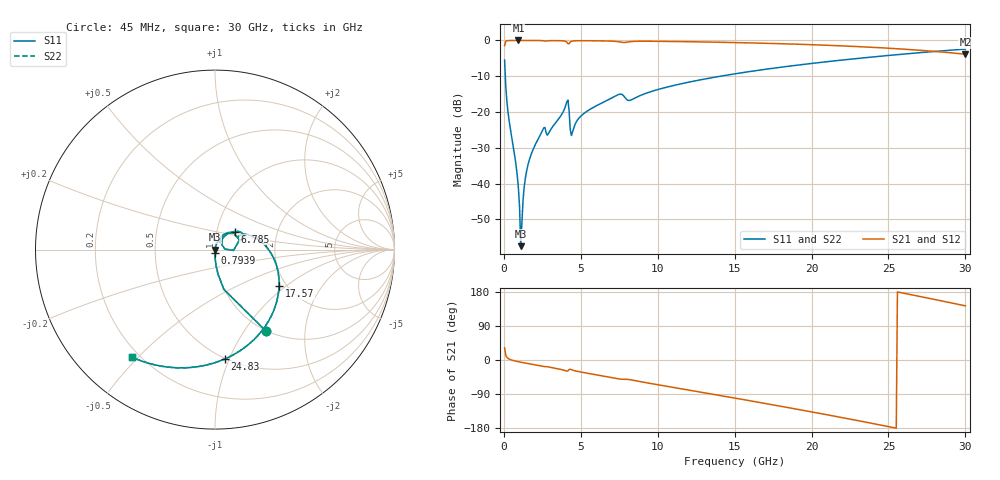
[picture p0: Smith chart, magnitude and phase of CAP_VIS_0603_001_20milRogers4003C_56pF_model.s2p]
! S-parameter model data by Modelithics Inc.  support@modelithics.com  813-866-6335  Tampa FL USA
! S-Parameter data specifications:
! Substrate: 20-mil Rogers 4003C, substrate thickness, H=0.508mm, Dielectric constant, Er=3.75
! PCB Mounting Pad Footprint: Pad width, PadW=0.90mm , Pad length, PadL=1.00mm , Pad gap, PadG (edge-to-edge)=1.00mm , Reference planes=3.0mm apart
! Created Wed Nov 18 13:29:34 2015
# hz S ma R 50
! 2 Port Network Data from SP1.SP block
! freq  magS11  angS11  magS21  angS21  magS12  angS12  magS22  angS22
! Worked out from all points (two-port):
!   401 points, 45 MHz to 30 GHz, reference 50 ohm
!   highest |S21| = -0.01 dB at 943.6 MHz (marker M1); lowest = -3.8 dB at 30 GHz (marker M2)
!   |S21| within 3 dB of the highest: start of sweep to 27.83 GHz
!   lowest |S11| = -57.5 dB at 1.093 GHz (marker M3), VSWR 1.00, Z = 50.1 - j0.1 ohm
!   |S11| at or under -10 dB: 90.84 MHz to 14.08 GHz (13.98 GHz wide, 197 % of centre)
!   |S22| runs from -57.5 to -2.4 dB; largest |S21 - S12| = 0
!   S11 on the Smith chart (normalised r, x): 45 MHz: 1.00, -1.25; 793.9 MHz: 1.00, -0.04; 6.785 GHz: 1.22, +0.25; 17.57 GHz: 1.83, -0.89; 24.83 GHz: 0.49, -0.96; 30 GHz: 0.17, -0.48
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4.5e7  0.5321 -58.1  0.8465 31.9  0.8465 31.9  0.5321 -58.1
3.4455e8  0.0742 -87.1  0.9966 2.4  0.9966 2.4  0.0742 -87.1
7.93875e8  0.01765 -90.5  0.9989 -3.2  0.9989 -3.2  0.01765 -90.5
9.4365e8  0.008555 -88.4  0.999 -4.6  0.999 -4.6  0.008555 -88.4
1.093425e9  0.001334 -48.4  0.9989 -5.8  0.9989 -5.8  0.001334 -48.4
1.2432e9  0.005846 72.7  0.9988 -7.0  0.9988 -7.0  0.005846 72.7
1.392975e9  0.01184 76.5  0.9987 -8.1  0.9987 -8.1  0.01184 76.5
1.617638e9  0.02017 76.7  0.9984 -9.8  0.9984 -9.8  0.02017 76.7
2.516288e9  0.05557 67.4  0.9925 -16.6  0.9925 -16.6  0.05557 67.4
2.965612e9  0.05326 65.0  0.9927 -18.9  0.9927 -18.9  0.05326 65.0
4.014038e9  0.123 50.8  0.9694 -28.4  0.9694 -28.4  0.123 50.8
4.463362e9  0.0528 44.8  0.9817 -26.7  0.9817 -26.7  0.0528 44.8
5.062462e9  0.0901 55.0  0.9911 -32.2  0.9911 -32.2  0.0901 55.0
6.784875e9  0.1482 42.8  0.982 -44.7  0.982 -44.7  0.1482 42.8
8.207738e9  0.1456 26.9  0.961 -52.0  0.961 -52.0  0.1456 26.9
1.007992e10  0.208 22.7  0.9717 -65.8  0.9717 -65.8  0.208 22.7
1.50225e10  0.3416 -11.3  0.934 -100.6  0.934 -100.6  0.3416 -11.3
1.756868e10  0.4104 -29.6  0.9055 -118.9  0.9055 -118.9  0.4104 -29.6
2.003996e10  0.4779 -47.8  0.8713 -137.2  0.8713 -137.2  0.4779 -47.8
2.483276e10  0.6118 -84.9  0.7822 -174.4  0.7822 -174.4  0.6118 -84.9
2.505742e10  0.6182 -86.7  0.7772 -176.2  0.7772 -176.2  0.6182 -86.7
3e10  0.7567 -127.5  0.6423 143.0  0.6423 143.0  0.7567 -127.5
